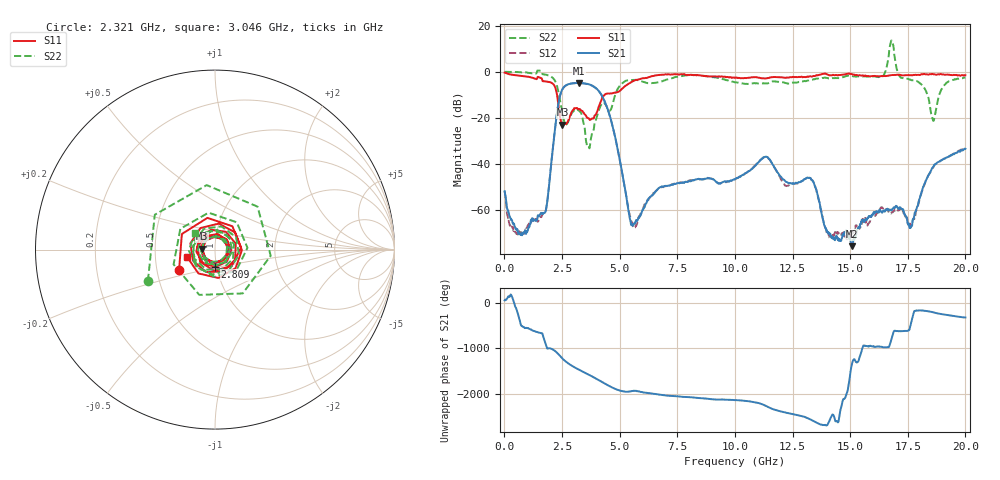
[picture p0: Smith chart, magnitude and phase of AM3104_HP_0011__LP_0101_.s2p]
!Created with skrf (http://scikit-rf.org).
# Hz S RI R 50.0
!freq ReS11 ImS11 ReS21 ImS21 ReS12 ImS12 ReS22 ImS22
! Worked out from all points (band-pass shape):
!   1601 points, 10 MHz to 20 GHz, reference 50 ohm
!   highest |S21| = -4.87 dB at 3.246 GHz (marker M1); lowest = -75.9 dB at 15.08 GHz (marker M2)
!   |S21| within 3 dB of the highest: 2.502 GHz to 4.05 GHz (1.548 GHz wide, 47.2 % of centre)
!   lowest |S11| = -23.0 dB at 2.521 GHz (marker M3), VSWR 1.15, Z = 43.4 + j0.44 ohm
!   |S11| at or under -10 dB: 2.283 GHz to 4.351 GHz (2.068 GHz wide, 62.4 % of centre)
!   |S22| runs from -33.3 to 13.6 dB; largest |S21 - S12| = 0.032
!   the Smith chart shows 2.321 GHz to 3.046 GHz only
!   S11 on the Smith chart (normalised r, x): 2.321 GHz: 0.65, -0.15; 2.809 GHz: 0.98, -0.19; 3.046 GHz: 0.73, -0.06
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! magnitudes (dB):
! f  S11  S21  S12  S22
! 10 MHz  -0.4  -52.0  -51.8  0.0
! 672.2 MHz  -1.7  -70.7  -69.7  -0.2
! 1.709 GHz  -4.2  -61.5  -61.4  -1.1
! 2.321 GHz  -12.8  -15.2  -15.2  -7.7
! 2.521 GHz  -23.0  -7.5  -7.6  -18.5
! 2.809 GHz  -20.3  -5.3  -5.4  -20.6
! 3.046 GHz  -15.9  -5.0  -5.0  -16.6
! 3.246 GHz  -16.4  -4.9  -5.0  -17.1
! 3.346 GHz  -16.9  -4.9  -5.0  -18.3
! 3.646 GHz  -20.2  -5.5  -5.6  -32.3
! 4.458 GHz  -9.5  -15.5  -15.6  -15.6
! 5.532 GHz  -4.3  -66.3  -65.5  -3.6
! 6.682 GHz  -1.4  -50.7  -50.8  -4.6
! 10.01 GHz  -2.7  -46.8  -46.8  -4.6
! 11.33 GHz  -2.9  -37.0  -37.3  -5.1
! 13.34 GHz  -2.1  -47.1  -47.0  -3.5
! 14.07 GHz  -1.4  -69.9  -71.0  -2.9
! 15.08 GHz  -1.0  -75.9  -69.7  -1.8
! 16.68 GHz  -1.6  -60.3  -61.1  7.2
! 17.63 GHz  -1.5  -67.8  -66.5  -3.5
! 18.6 GHz  -1.1  -41.5  -41.7  -21.2
! 20 GHz  -1.5  -33.5  -33.2  -2.5
